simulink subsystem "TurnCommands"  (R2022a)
settings: Solver=VariableStepAuto  StartTime=0.0  StopTime=10.0  RelTol=1e-3
undefined symbols (not defined in the file or in its folder): Euler_0
libraries: slpidlib x3, simulink x3

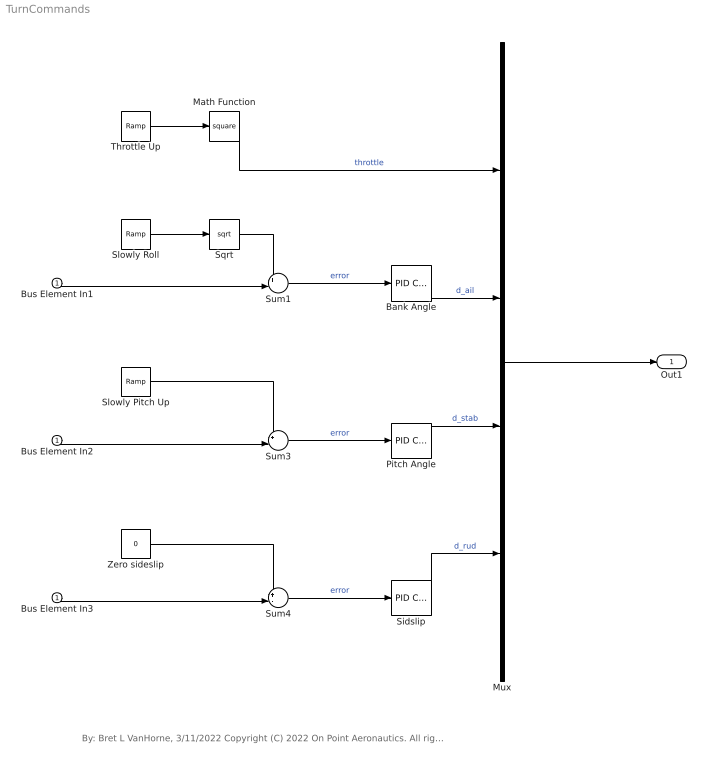
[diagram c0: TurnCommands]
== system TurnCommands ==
  note: By: Bret L VanHorne, 3/11/2022 Copyright (C) 2022 On Point Aeronautics. All rights reserved.
  Bus Element In1 : Inport
  Bus Element In2 : Inport
  Bus Element In3 : Inport
  Bank Angle : slpidlib/PID Controller  Controller=PID  Form=Parallel  TimeDomain=Continuous-time  UseExternalTs=off  SampleTime=-1  IntegratorMethod=Forward Euler  FilterMethod=Forward Euler  ControllerParametersSource=internal  P=-4.5  I=0  UseKiTs=off  D=-3  N=100  UseFilter=on  TunerSelectOption=Transfer Function Based (PID Tuner App)  InitialConditionSource=internal  InitialConditionForIntegrator=0  InitialConditionForFilter=0  DifferentiatorICPrevScaledInput=0  ExternalReset=none  TrackingMode=off  Kt=1  LimitOutput=off  SatLimitsSource=internal  UpperSaturationLimit=inf  LowerSaturationLimit=-inf  LinearizeAsGain=on  AntiWindupMode=none  Kb=1  POutMin=[]  POutMax=[]  IOutMin=[]  IOutMax=[]  DOutMin=[]  DOutMax=[]  NOutMin=[]  NOutMax=[]  SumOutMin=[]  SumOutMax=[]  SaturationOutMin=[]  SaturationOutMax=[]  PParamMin=[]  PParamMax=[]  IParamMin=[]  IParamMax=[]  DParamMin=[]  DParamMax=[]  NParamMin=[]  NParamMax=[]  KbParamMin=[]  KbParamMax=[]  KtParamMin=[]  KtParamMax=[]  KbOutMin=[]  KbOutMax=[]  KtOutMin=[]  KtOutMax=[]  IntegratorOutMin=[]  IntegratorOutMax=[]  FilterOutMin=[]  FilterOutMax=[]  SumI1OutMin=[]  SumI1OutMax=[]  SumI2OutMin=[]  SumI2OutMax=[]  SumI3OutMin=[]  SumI3OutMax=[]  SumI4OutMin=[]  SumI4OutMax=[]  SumDOutMin=[]  SumDOutMax=[]  DifferentiatorOutMin=[]  DifferentiatorOutMax=[]  FilterDiffOutCoefMin=[]  FilterDiffOutCoefMax=[]  ReciprocalOutMin=[]  ReciprocalOutMax=[]  SumDenOutMin=[]  SumDenOutMax=[]  SumNumOutMin=[]  SumNumOutMax=[]  DivideOutMin=[]  DivideOutMax=[]  UdiffTsProdOutMin=[]  UdiffTsProdOutMax=[]  NTsProdOutMin=[]  NTsProdOutMax=[]  UintegralTsProdOutMin=[]  UintegralTsProdOutMax=[]  UngainTsProdOutMin=[]  UngainTsProdOutMax=[]  IntegratorContinuousStateAttributes=''  IntegratorStateMustResolveToSignalObject=off  IntegratorRTWStateStorageClass=Auto  FilterContinuousStateAttributes=''  FilterStateMustResolveToSignalObject=off  FilterRTWStateStorageClass=Auto  ParallelPVariant=InternalParameters  IdealPVariant=Disabled  IVariant=InternalParameters  DVariant=InternalParameters  IntegratorVariant=Continuous  SatVariant=Disabled  AWVariant=Passthrough  PCopyVariant=Disabled  TRVariant=Disabled  FdbkBlocksVariant=Forward  IdealPFdbkVariant=Disabled  SatFdbkVariant=Disabled  DerivativeFilterVariant=ContFilter  NVariant=InternalParameters  NCopyVariant=Disabled  FilterICVariant=InternalICsFilter  IntegratorICVariant=InternalICs  ExternalResetVariant=Disabled  TRSumVariant=Passthrough  SumFdbkVariant=Disabled  SumVariant=Sum_PID  TsampFilterVariant=InternalTs  TsampNgainVariant=Passthrough  TsampIntegralVariant=Passthrough  ExternalSaturationOutDataTypeStr=Inherit: Same as second input  aMode=0
  Math Function : Math  Operator=square
  Mux : Mux
  Pitch Angle : slpidlib/PID Controller  Controller=PID  Form=Parallel  TimeDomain=Continuous-time  UseExternalTs=off  SampleTime=-1  IntegratorMethod=Forward Euler  FilterMethod=Forward Euler  ControllerParametersSource=internal  P=-35  I=-1  UseKiTs=off  D=-10  N=100  UseFilter=on  TunerSelectOption=Transfer Function Based (PID Tuner App)  InitialConditionSource=internal  InitialConditionForIntegrator=0  InitialConditionForFilter=0  DifferentiatorICPrevScaledInput=0  ExternalReset=none  TrackingMode=off  Kt=1  LimitOutput=off  SatLimitsSource=internal  UpperSaturationLimit=inf  LowerSaturationLimit=-inf  LinearizeAsGain=on  AntiWindupMode=none  Kb=1  POutMin=[]  POutMax=[]  IOutMin=[]  IOutMax=[]  DOutMin=[]  DOutMax=[]  NOutMin=[]  NOutMax=[]  SumOutMin=[]  SumOutMax=[]  SaturationOutMin=[]  SaturationOutMax=[]  PParamMin=[]  PParamMax=[]  IParamMin=[]  IParamMax=[]  DParamMin=[]  DParamMax=[]  NParamMin=[]  NParamMax=[]  KbParamMin=[]  KbParamMax=[]  KtParamMin=[]  KtParamMax=[]  KbOutMin=[]  KbOutMax=[]  KtOutMin=[]  KtOutMax=[]  IntegratorOutMin=[]  IntegratorOutMax=[]  FilterOutMin=[]  FilterOutMax=[]  SumI1OutMin=[]  SumI1OutMax=[]  SumI2OutMin=[]  SumI2OutMax=[]  SumI3OutMin=[]  SumI3OutMax=[]  SumI4OutMin=[]  SumI4OutMax=[]  SumDOutMin=[]  SumDOutMax=[]  DifferentiatorOutMin=[]  DifferentiatorOutMax=[]  FilterDiffOutCoefMin=[]  FilterDiffOutCoefMax=[]  ReciprocalOutMin=[]  ReciprocalOutMax=[]  SumDenOutMin=[]  SumDenOutMax=[]  SumNumOutMin=[]  SumNumOutMax=[]  DivideOutMin=[]  DivideOutMax=[]  UdiffTsProdOutMin=[]  UdiffTsProdOutMax=[]  NTsProdOutMin=[]  NTsProdOutMax=[]  UintegralTsProdOutMin=[]  UintegralTsProdOutMax=[]  UngainTsProdOutMin=[]  UngainTsProdOutMax=[]  IntegratorContinuousStateAttributes=''  IntegratorStateMustResolveToSignalObject=off  IntegratorRTWStateStorageClass=Auto  FilterContinuousStateAttributes=''  FilterStateMustResolveToSignalObject=off  FilterRTWStateStorageClass=Auto  ParallelPVariant=InternalParameters  IdealPVariant=Disabled  IVariant=InternalParameters  DVariant=InternalParameters  IntegratorVariant=Continuous  SatVariant=Disabled  AWVariant=Passthrough  PCopyVariant=Disabled  TRVariant=Disabled  FdbkBlocksVariant=Forward  IdealPFdbkVariant=Disabled  SatFdbkVariant=Disabled  DerivativeFilterVariant=ContFilter  NVariant=InternalParameters  NCopyVariant=Disabled  FilterICVariant=InternalICsFilter  IntegratorICVariant=InternalICs  ExternalResetVariant=Disabled  TRSumVariant=Passthrough  SumFdbkVariant=Disabled  SumVariant=Sum_PID  TsampFilterVariant=InternalTs  TsampNgainVariant=Passthrough  TsampIntegralVariant=Passthrough  ExternalSaturationOutDataTypeStr=Inherit: Same as second input  aMode=0
  Sidslip : slpidlib/PID Controller  Controller=PID  Form=Parallel  TimeDomain=Continuous-time  UseExternalTs=off  SampleTime=-1  IntegratorMethod=Forward Euler  FilterMethod=Forward Euler  ControllerParametersSource=internal  P=50  I=0  UseKiTs=off  D=15  N=100  UseFilter=on  TunerSelectOption=Transfer Function Based (PID Tuner App)  InitialConditionSource=internal  InitialConditionForIntegrator=0  InitialConditionForFilter=0  DifferentiatorICPrevScaledInput=0  ExternalReset=none  TrackingMode=off  Kt=1  LimitOutput=off  SatLimitsSource=internal  UpperSaturationLimit=inf  LowerSaturationLimit=-inf  LinearizeAsGain=on  AntiWindupMode=none  Kb=1  POutMin=[]  POutMax=[]  IOutMin=[]  IOutMax=[]  DOutMin=[]  DOutMax=[]  NOutMin=[]  NOutMax=[]  SumOutMin=[]  SumOutMax=[]  SaturationOutMin=[]  SaturationOutMax=[]  PParamMin=[]  PParamMax=[]  IParamMin=[]  IParamMax=[]  DParamMin=[]  DParamMax=[]  NParamMin=[]  NParamMax=[]  KbParamMin=[]  KbParamMax=[]  KtParamMin=[]  KtParamMax=[]  KbOutMin=[]  KbOutMax=[]  KtOutMin=[]  KtOutMax=[]  IntegratorOutMin=[]  IntegratorOutMax=[]  FilterOutMin=[]  FilterOutMax=[]  SumI1OutMin=[]  SumI1OutMax=[]  SumI2OutMin=[]  SumI2OutMax=[]  SumI3OutMin=[]  SumI3OutMax=[]  SumI4OutMin=[]  SumI4OutMax=[]  SumDOutMin=[]  SumDOutMax=[]  DifferentiatorOutMin=[]  DifferentiatorOutMax=[]  FilterDiffOutCoefMin=[]  FilterDiffOutCoefMax=[]  ReciprocalOutMin=[]  ReciprocalOutMax=[]  SumDenOutMin=[]  SumDenOutMax=[]  SumNumOutMin=[]  SumNumOutMax=[]  DivideOutMin=[]  DivideOutMax=[]  UdiffTsProdOutMin=[]  UdiffTsProdOutMax=[]  NTsProdOutMin=[]  NTsProdOutMax=[]  UintegralTsProdOutMin=[]  UintegralTsProdOutMax=[]  UngainTsProdOutMin=[]  UngainTsProdOutMax=[]  IntegratorContinuousStateAttributes=''  IntegratorStateMustResolveToSignalObject=off  IntegratorRTWStateStorageClass=Auto  FilterContinuousStateAttributes=''  FilterStateMustResolveToSignalObject=off  FilterRTWStateStorageClass=Auto  ParallelPVariant=InternalParameters  IdealPVariant=Disabled  IVariant=InternalParameters  DVariant=InternalParameters  IntegratorVariant=Continuous  SatVariant=Disabled  AWVariant=Passthrough  PCopyVariant=Disabled  TRVariant=Disabled  FdbkBlocksVariant=Forward  IdealPFdbkVariant=Disabled  SatFdbkVariant=Disabled  DerivativeFilterVariant=ContFilter  NVariant=InternalParameters  NCopyVariant=Disabled  FilterICVariant=InternalICsFilter  IntegratorICVariant=InternalICs  ExternalResetVariant=Disabled  TRSumVariant=Passthrough  SumFdbkVariant=Disabled  SumVariant=Sum_PID  TsampFilterVariant=InternalTs  TsampNgainVariant=Passthrough  TsampIntegralVariant=Passthrough  ExternalSaturationOutDataTypeStr=Inherit: Same as second input  aMode=0
  Slowly Pitch Up : simulink/Sources/Ramp  slope=.0025  start=10  InitialOutput=Euler_0(2)
  Slowly Roll : simulink/Sources/Ramp  slope=deg2rad(2)  start=10  InitialOutput=0
  Sqrt : Sqrt
  Sum1 : Sum  Inputs=+-|
  Sum3 : Sum  Inputs=+-|
  Sum4 : Sum  Inputs=+-|
  Throttle Up : simulink/Sources/Ramp  slope=.014  start=10  InitialOutput=0
  Zero sideslip : Constant  Value=0
  Out1 : Outport
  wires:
  Throttle Up/1 -> Math Function/1
  Slowly Roll/1 -> Sqrt/1
  Sum4/1 -> Sidslip/1  "error"
  Bank Angle/1 -> Mux/2  "d_ail"
  Sum3/1 -> Pitch Angle/1  "error"
  Zero sideslip/1 -> Sum4/1
  Sum1/1 -> Bank Angle/1  "error"
  Bus Element In2/1 -> Sum3/2
  Sidslip/1 -> Mux/4  "d_rud"
  Bus Element In3/1 -> Sum4/2
  Pitch Angle/1 -> Mux/3  "d_stab"
  Mux/1 -> Out1/1
  Bus Element In1/1 -> Sum1/2
  Sqrt/1 -> Sum1/1
  Slowly Pitch Up/1 -> Sum3/1
  Math Function/1 -> Mux/1  "throttle"
